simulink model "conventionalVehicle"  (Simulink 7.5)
settings: Solver=ode45  StartTime=0.0  StopTime=Tfinal  RelTol=1e-3
InitFcn:
  | t_Start=tic;
StopFcn:
  | t_elapsed=toc(t_Start);
  | fuel_cons=(1000*(fueltank_simple1_std(end,1)/fueltank_simple1_std(end,3)))/(chassis_simple4_std(end,2)/100000);
  | 
  | disp(' ')
  | disp(['Time Elapsed: ' num2str(round(100*t_elapsed)/100) 's'])
  | disp(['Fuel Consumption: ' num2str(round(1000*fuel_cons)/1000) 'L/100km'])
undefined symbols (not defined in the file or in its folder): computed_mass, DC, levelinit
libraries: simulink x10, simulink_extras x2
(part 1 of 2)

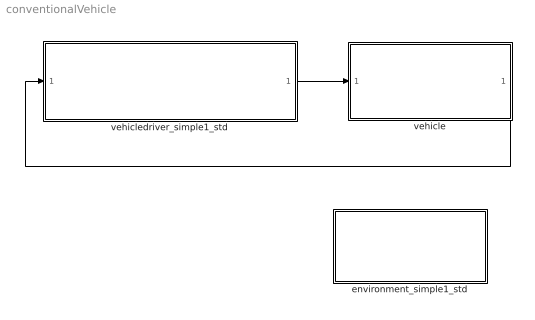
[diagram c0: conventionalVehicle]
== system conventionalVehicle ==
  environment_simple1_std : Subsystem  mask{Tamb=300, Pamb=101300}
      mask prompts: Tamb "Ambient Temperature [K]"; Pamb "Ambient Pressure [Pa]"
      mask help: Environment settings
  vehicle : Subsystem
  vehicledriver_simple1_std : Subsystem  mask{Kp_driver=0.5, Ki_driver=0.05, clutchtime=0.5, manualFlag=1, nog=5}
      mask prompts: Kp_driver "Proportional Gain"; Ki_driver "Integral Gain"; clutchtime "Gear change time"; manualFlag "Manual or automatic gearchange?"; nog "Number of gears"
      mask help: Driver model
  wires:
  vehicledriver_simple1_std/1(driver cmd out) -> vehicle/1(In1)
  vehicle/1(Out1) -> vehicledriver_simple1_std/1(vehicle fb in)

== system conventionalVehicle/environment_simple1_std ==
  Clock : Clock
  Constant : Constant  Value=Tamb  OutDataType=sfix(16)  OutScaling=2^0
  Constant1 : Constant  Value=Pamb  OutDataType=sfix(16)  OutScaling=2^0
  Mux : Mux  Inputs=3
  Mux1 : Mux  Inputs=3
  Mux2 : Mux  Inputs=5
  To Workspace : ToWorkspace  VariableName=environment_simple1_std  SampleTime=-1  SaveFormat=Array
  fric_time : Lookup  InputValues=DC.time  Table=DC.fric  OutDataType=sfix(16)  OutScaling=2^0
  gear_time : Lookup  InputValues=DC.time  Table=DC.gearnr  OutDataType=sfix(16)  OutScaling=2^0
  slope_x_time : Lookup  InputValues=DC.time  Table=DC.slope_x  OutDataType=sfix(16)  OutScaling=2^0
  slope_y_time : Lookup  InputValues=DC.time  Table=DC.slope_y  OutDataType=sfix(16)  OutScaling=2^0
  speed_ref_time : Lookup  InputValues=DC.time  Table=DC.speed  OutDataType=sfix(16)  OutScaling=2^0
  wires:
  Constant1/1 -> Mux/2, Mux2/5
  Constant/1 -> Mux/1, Mux2/4
  Mux/1 -> To Workspace/1
  Clock/1 -> speed_ref_time/1, gear_time/1, slope_x_time/1, slope_y_time/1, fric_time/1, Mux/3, Mux1/3  "t"
  Mux1/1 -> [drivecycle]
  gear_time/1 -> Mux1/2
  slope_x_time/1 -> Mux2/1
  slope_y_time/1 -> Mux2/2
  fric_time/1 -> Mux2/3
  Mux2/1 -> [environment]
  speed_ref_time/1 -> Mux1/1

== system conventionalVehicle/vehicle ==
  In1 : Inport  OutDataType=sfix(16)  OutScaling=2^0
  Bus Creator : BusCreator  Inputs=3
  Bus Creator1 : BusCreator  Inputs=1
  Bus Selector : BusSelector  OutputSignals=ice,clutch,gearbox,chassis
  Ground : Ground
  Terminator : Terminator
  chassis_simple4_std : Subsystem  InitFcn=computed_mass=calc_total_mass;
  clutch_simple1_std : Subsystem
  controller_conventional1_std : Subsystem  mask{pedalmap_pedal=[0 1], idleSpeed=78.5, pedalmap_speed=[0 700], pedalmap_torqueref=[0 0;350 350], maxTorque=400, maxBrakeTorque=40000}
      mask prompts: pedalmap_pedal "Pedal Map: Input pedalvector"; idleSpeed "Idle speed (rad/s)"; pedalmap_speed "Pedal Map: Input speedvector"; pedalmap_torqueref "Pedal Map: PedalMap (torqueref)"; maxTorque "Maximum torque reference (Nm)"; maxBrakeTorque "Maximum brake torque (Nm)"
      mask help: Main Controller
  engine_scalable1_std : Subsystem
  fueltank_simple1_std : Subsystem  mask{tanksize=68, level=100, fueldensity=737.2, Hf=44.6}
      mask prompts: tanksize "Size of fuel tank  [l]"; level "Level in tank [%]"; fueldensity "Fuel density [kg/m3]"; Hf "Specific Calorific Value [MJ/kg]"
      mask help: This is an ideal internal combustion engine component
  gearbox_manual1_std : Subsystem
  Out1 : Outport  OutDataType=sfix(16)  OutScaling=2^0
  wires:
  In1/1 -> controller_conventional1_std/1(driver cmd in)
  controller_conventional1_std/1(vehicle fb out) -> Out1/1
  gearbox_manual1_std/2(mech power out [Nm]) -> chassis_simple4_std/2(mech in [Nm])
  clutch_simple1_std/1(mech power out [Nm]) -> gearbox_manual1_std/2(mech power in [Nm])
  clutch_simple1_std/2(mech fb out [rad/s]) -> engine_scalable1_std/3(mech fb in [rad/s])
  engine_scalable1_std/2(mech out [Nm]) -> clutch_simple1_std/2(mech power in [Nm])
  fueltank_simple1_std/1(chem SCV out [MJ/kg]) -> engine_scalable1_std/2(chem SCV in [MJ/kg])
  engine_scalable1_std/3(chem fb out [kg/s]) -> fueltank_simple1_std/1(chem fb in [kg/s])
  gearbox_manual1_std/3(mech fb out [rad/s]) -> clutch_simple1_std/3(mech fb in [rad/s])
  chassis_simple4_std/2(mech fb out [rad/s]) -> gearbox_manual1_std/3(mech fb in [rad/s])
  Bus Creator/1 -> controller_conventional1_std/2(sensor in)
  controller_conventional1_std/2(cmd out) -> Bus Selector/1
  engine_scalable1_std/1(sensor out) -> Bus Creator/1
  gearbox_manual1_std/1(sensor out) -> Bus Creator/2
  chassis_simple4_std/1(sensor out) -> Bus Creator/3
  Bus Selector/1 -> engine_scalable1_std/1(cmd)  "<ice>"
  Bus Selector/2 -> clutch_simple1_std/1(cmd)  "<clutch>"
  Bus Selector/3 -> gearbox_manual1_std/1(cmd)  "<gearbox>"
  Bus Selector/4 -> chassis_simple4_std/1(cmd)  "<chassis>"
  chassis_simple4_std/3(el fb out [A]) -> Terminator/1
  Bus Creator1/1 -> chassis_simple4_std/3(el in [V])
  Ground/1 -> Bus Creator1/1  "voltage [V]"

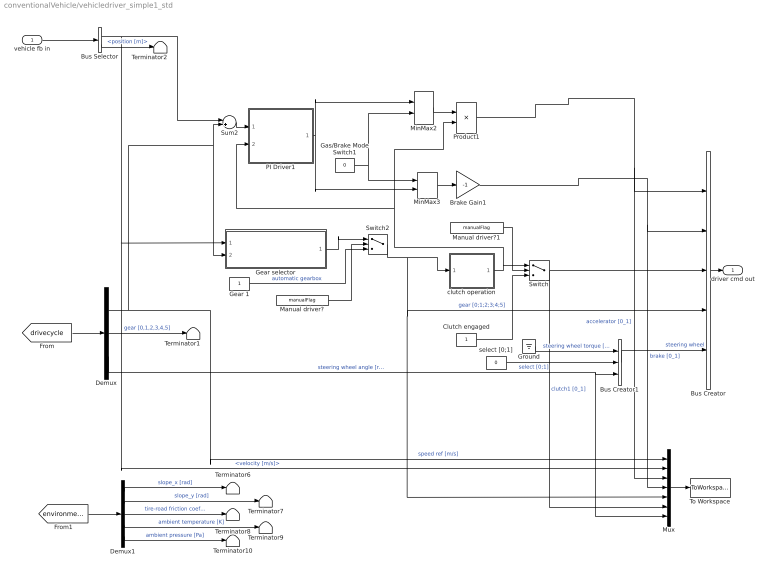
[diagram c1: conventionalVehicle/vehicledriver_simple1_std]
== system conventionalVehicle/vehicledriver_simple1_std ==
  vehicle fb in : Inport  OutDataType=sfix(16)  OutScaling=2^0
  Brake Gain1 : Gain  Gain=-1  ParameterDataType=sfix(16)  ParameterScaling=2^0  OutDataType=sfix(16)  OutScaling=2^0
  Bus Creator : BusCreator  Inputs=5
  Bus Creator1 : BusCreator  Inputs=3
  Bus Selector : BusSelector  OutputSignals=chassis.velocity [m/s],chassis.position [m]
  Clutch engaged : Constant  OutDataType=sfix(16)  OutScaling=2^0
  Demux : Demux  Outputs=3
  Demux1 : Demux  Outputs=5
  Gas/Brake Mode Switch1 : Constant  Value=0  OutDataType=sfix(16)  OutScaling=2^0
  Gear 1 : Constant  OutDataType=sfix(16)  OutScaling=2^0
  Gear selector : Subsystem
  Ground : Ground
  Manual driver? : Constant  Value=manualFlag  OutDataType=sfix(16)  OutScaling=2^0
  Manual driver?1 : Constant  Value=manualFlag  OutDataType=sfix(16)  OutScaling=2^0
  MinMax2 : MinMax  Function=max  Inputs=2  OutDataType=sfix(16)  OutScaling=2^0
  MinMax3 : MinMax  Inputs=2  OutDataType=sfix(16)  OutScaling=2^0
  Mux : Mux  Inputs=7
  PI Driver1 : Subsystem
  Product1 : Product  OutDataType=sfix(16)  OutScaling=2^0
  Sum2 : Sum  Inputs=-+  OutDataType=sfix(16)  OutScaling=2^0
  Switch : Switch  Criteria=u2 > Threshold
  Switch2 : Switch  Criteria=u2 > Threshold
  Terminator{1..2,6..10} (7 alike) : Terminator
  To Workspace : ToWorkspace  VariableName=vehicledriver_simple1_std  SampleTime=-1  SaveFormat=Array
  clutch operation : Subsystem
  select [0;1] : Constant  Value=0  OutDataType=sfix(16)  OutScaling=2^0
  driver cmd out : Outport  OutDataType=sfix(16)  OutScaling=2^0
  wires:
  Bus Selector/2 -> Terminator2/1  "<position [m]>"
  Bus Selector/1 -> Mux/2, Gear selector/1(Speed [m/s]), Sum2/1  "<velocity [m/s]>"
  vehicle fb in/1 -> Bus Selector/1
  Sum2/1 -> PI Driver1/1(PI input)
  Brake Gain1/1 -> Mux/4, Bus Creator/2  "brake [0_1]"
  PI Driver1/1(PI out) -> MinMax2/1, MinMax3/2
  MinMax3/1 -> Brake Gain1/1
  Gas/Brake Mode Switch1/1 -> MinMax2/2, MinMax3/1
  MinMax2/1 -> Product1/1
  Product1/1 -> Mux/3, Bus Creator/1  "accelerator [0_1]"
  Switch/1 -> Mux/6, Bus Creator/3  "clutch1 [0_1]"
  clutch operation/1(Clutch) -> Product1/2, PI Driver1/2(PI reset), Switch/1
  Switch2/1 -> Mux/5, Bus Creator/4, clutch operation/1(Gear)  "gear [0;1;2;3;4;5]"
  Bus Creator1/1 -> Bus Creator/5  "steering wheel"
  Mux/1 -> To Workspace/1
  Ground/1 -> Bus Creator1/1  "steering wheel torque [Nm]"
  Bus Creator/1 -> driver cmd out/1
  Manual driver?1/1 -> Switch/2
  Demux1/2 -> Terminator7/1  "slope_y [rad]"
  [environment] -> Demux1/1
  Demux1/3 -> Terminator8/1  "tire-road friction coefficient [-]"
  Demux1/1 -> Terminator6/1  "slope_x [rad]"
  Demux1/4 -> Terminator9/1  "ambient temperature [K]"
  Demux1/5 -> Terminator10/1  "ambient pressure [Pa]"
  Demux/2 -> Terminator1/1  "gear [0,1,2,3,4,5]"
  [drivecycle] -> Demux/1
  Demux/3 -> Bus Creator1/3, Mux/7  "steering wheel angle [rad]"
  Demux/1 -> Mux/1, Sum2/2, Gear selector/2(Speed ref [m/s])  "speed ref [m/s]"
  select [0;1]/1 -> Bus Creator1/2  "select [0;1]"
  Gear 1/1 -> Switch2/3  "automatic gearbox"
  Gear selector/1(Gear [0,1,2,3,4,5]) -> Switch2/1
  Manual driver?/1 -> Switch2/2
  Clutch engaged/1 -> Switch/3

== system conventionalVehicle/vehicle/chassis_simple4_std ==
  cmd : Inport  OutDataType=sfix(16)  OutScaling=2^0
  mech in [Nm] : Inport  Port=2  OutDataType=sfix(16)  OutScaling=2^0
  el in [V] : Inport  Port=3  OutDataType=sfix(16)  OutScaling=2^0
  chassis : Subsystem  mask{mass=??, nop=1, passengerweight=0, cargo=0, w_init=0, tirespec='215/45R16', e=0.01, Cd=0.3, Af=1.9, rho=1.29, finalgear=1}
      mask prompts: mass "Chassis Mass [kg]"; nop "Number of passengers"; passengerweight "Weight of avg. passenger (kg)"; cargo "Cargo load (kg)"; w_init "Initial velocity [rad/s]"; tirespec "Tire specification (ex: '205/55R16')"; e "Rolling resistance coeff rear"; Cd "Air resistance cd (-)"; Af "Air resistance frontal area (m2)"; rho "Air density (kg/m3)"; finalgear "Final gear"
      mask help: Chassis model template
      mask init:
      | r=tireradius(tirespec);
  local controller : Subsystem
  sensor out : Outport  OutDataType=sfix(16)  OutScaling=2^0
  mech fb out [rad/s] : Outport  Port=2  OutDataType=sfix(16)  OutScaling=2^0
  el fb out [A] : Outport  Port=3  OutDataType=sfix(16)  OutScaling=2^0
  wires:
  local controller/2(ctrl) -> chassis/1(ctrl)
  chassis/2(mech fb out [rad/s]) -> mech fb out [rad/s]/1
  mech in [Nm]/1 -> chassis/2(mech in [Nm])
  chassis/1(sensor out) -> local controller/2(sensor in)
  local controller/1(sensor out) -> sensor out/1
  cmd/1 -> local controller/1(cmd in)
  el in [V]/1 -> chassis/3(el in [V])
  chassis/3(el fb out [A]) -> el fb out [A]/1

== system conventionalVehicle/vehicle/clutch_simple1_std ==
  cmd : Inport  OutDataType=sfix(16)  OutScaling=2^0
  mech power in [Nm] : Inport  Port=2  OutDataType=sfix(16)  OutScaling=2^0
  mech fb in [rad/s] : Inport  Port=3  OutDataType=sfix(16)  OutScaling=2^0
  clutch : Subsystem  mask{mass=0, inertia=0.25, max_torque=500}
      mask prompts: mass "Component mass (kg)"; inertia "Clutch inertia (kgm^2)"; max_torque "Maximum clutch torque (Nm)"
  local controller : Subsystem
  mech power out [Nm] : Outport  OutDataType=sfix(16)  OutScaling=2^0
  mech fb out [rad/s] : Outport  Port=2  OutDataType=sfix(16)  OutScaling=2^0
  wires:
  mech power in [Nm]/1 -> clutch/2(mech power in [Nm])
  clutch/2(mech power out [Nm]) -> mech power out [Nm]/1
  mech fb in [rad/s]/1 -> clutch/3(mech fb in [rad/s])
  clutch/3(mech fb out [rad/s]) -> mech fb out [rad/s]/1
  cmd/1 -> local controller/1(cmd)
  local controller/1(ctrl) -> clutch/1(ctrl)
  clutch/1(sensor out) -> local controller/2(sensor in)

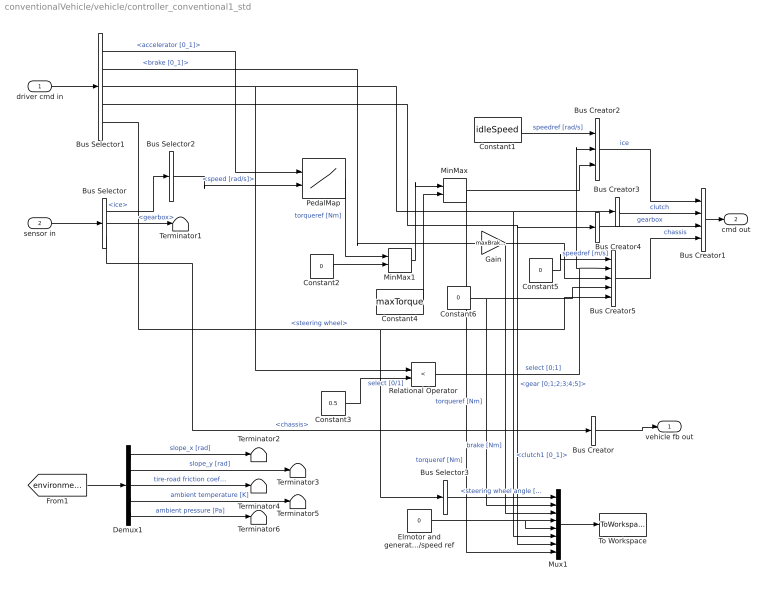
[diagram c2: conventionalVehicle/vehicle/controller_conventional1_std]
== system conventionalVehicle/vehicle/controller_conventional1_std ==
  driver cmd in : Inport  OutDataType=sfix(16)  OutScaling=2^0
  sensor in : Inport  Port=2  OutDataType=sfix(16)  OutScaling=2^0
  Bus Creator : BusCreator  Inputs=1
  Bus Creator1 : BusCreator
  Bus Creator2 : BusCreator  Inputs=3
  Bus Creator3 : BusCreator  Inputs=1
  Bus Creator4 : BusCreator  Inputs=1
  Bus Creator5 : BusCreator  Inputs=5
  Bus Selector : BusSelector  OutputSignals=ice,gearbox,chassis
  Bus Selector1 : BusSelector  OutputSignals=accelerator [0_1],brake [0_1],clutch1 [0_1],gear [0;1;2;3;4;5],steering wheel
  Bus Selector2 : BusSelector  OutputSignals=speed [rad/s]
  Bus Selector3 : BusSelector  OutputSignals=steering wheel angle [rad]
  Constant1 : Constant  Value=idleSpeed  OutDataType=sfix(16)  OutScaling=2^0
  Constant2 : Constant  Value=0  OutDataType=sfix(16)  OutScaling=2^0
  Constant3 : Constant  Value=0.5  OutDataType=sfix(16)  OutScaling=2^0
  Constant4 : Constant  Value=maxTorque  OutDataType=sfix(16)  OutScaling=2^0
  Constant5 : Constant  Value=0  OutDataType=sfix(16)  OutScaling=2^0
  Constant6 : Constant  Value=0  OutDataType=sfix(16)  OutScaling=2^0
  Demux1 : Demux  Outputs=5
  Elmotor and generator torque/speed ref : Constant  Value=0  OutDataType=sfix(16)  OutScaling=2^0
  Gain : Gain  Gain=maxBrakeTorque  ParameterDataType=sfix(16)  ParameterScaling=2^0  OutDataType=sfix(16)  OutScaling=2^0
  MinMax : MinMax  Inputs=2  OutDataType=sfix(16)  OutScaling=2^0
  MinMax1 : MinMax  Function=max  Inputs=2  OutDataType=sfix(16)  OutScaling=2^0
  Mux1 : Mux  Inputs=8
  PedalMap : Lookup2D  RowIndex=pedalmap_pedal  ColumnIndex=pedalmap_speed  Table=pedalmap_torqueref  OutDataType=sfix(16)  OutScaling=2^0
  Relational Operator : RelationalOperator  Operator=<
  Terminator{1..6} (6 alike) : Terminator
  To Workspace : ToWorkspace  VariableName=controller_conventional1_std  SampleTime=-1  SaveFormat=Array
  vehicle fb out : Outport  OutDataType=sfix(16)  OutScaling=2^0
  cmd out : Outport  Port=2  OutDataType=sfix(16)  OutScaling=2^0
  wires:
  Bus Selector2/1 -> PedalMap/2  "<speed [rad/s]>"
  Relational Operator/1 -> Bus Creator2/2, Bus Creator5/2  "select [0;1]"
  MinMax1/1 -> MinMax/1
  Constant4/1 -> MinMax/2
  Constant2/1 -> MinMax1/2
  PedalMap/1 -> MinMax1/1  "torqueref [Nm]"
  Constant3/1 -> Relational Operator/2  "select [0/1]"
  MinMax/1 -> Bus Creator2/3, Mux1/8  "torqueref [Nm]"
  Constant1/1 -> Bus Creator2/1  "speedref [rad/s]"
  Bus Creator2/1 -> Bus Creator1/1  "ice"
  Bus Creator1/1 -> cmd out/1
  Bus Creator/1 -> vehicle fb out/1
  Bus Selector/1 -> Bus Selector2/1  "<ice>"
  Bus Selector/2 -> Terminator1/1  "<gearbox>"
  Bus Selector/3 -> Bus Creator/1  "<chassis>"
  sensor in/1 -> Bus Selector/1
  driver cmd in/1 -> Bus Selector1/1
  Bus Creator3/1 -> Bus Creator1/2  "clutch"
  Bus Creator4/1 -> Bus Creator1/3  "gearbox"
  Gain/1 -> Bus Creator5/3, Mux1/3  "brake [Nm]"
  Bus Creator5/1 -> Bus Creator1/4  "chassis"
  Bus Selector1/1 -> PedalMap/1  "<accelerator [0_1]>"
  Bus Selector1/2 -> Gain/1  "<brake [0_1]>"
  Bus Selector1/3 -> Relational Operator/1, Bus Creator3/1, Mux1/6  "<clutch1 [0_1]>"
  Bus Selector1/5 -> Bus Creator5/5, Bus Selector3/1  "<steering wheel>"
  Bus Selector1/4 -> Bus Creator4/1, Mux1/7  "<gear [0;1;2;3;4;5]>"
  Mux1/1 -> To Workspace/1
  Bus Selector3/1 -> Mux1/1  "<steering wheel angle [rad]>"
  Constant5/1 -> Bus Creator5/1  "speedref [m/s]"
  Constant6/1 -> Bus Creator5/4, Mux1/2  "torqueref [Nm]"
  Elmotor and generator torque/speed ref/1 -> Mux1/4, Mux1/5
  Demux1/2 -> Terminator3/1  "slope_y [rad]"
  [environment] -> Demux1/1
  Demux1/3 -> Terminator4/1  "tire-road friction coefficient [-]"
  Demux1/1 -> Terminator2/1  "slope_x [rad]"
  Demux1/4 -> Terminator5/1  "ambient temperature [K]"
  Demux1/5 -> Terminator6/1  "ambient pressure [Pa]"

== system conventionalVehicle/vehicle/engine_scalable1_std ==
  cmd : Inport  OutDataType=sfix(16)  OutScaling=2^0
  chem SCV in [MJ/kg] : Inport  Port=2  OutDataType=sfix(16)  OutScaling=2^0
  mech fb in [rad/s] : Inport  Port=3  OutDataType=sfix(16)  OutScaling=2^0
  Model Info1 : simulink/Model-Wide Utilities/Model Info  SystemSampleTime=-1  InitialBlockCM=None  BlockCM=None  Frame=on  DisplayStringWithTags=This model level is fixed. Place parameters in the subsystem masks, not on the top level.  HorizontalTextAlignment=Left  LeftAlignmentValue=0.02  SourceBlockDiagram=conventionalVehicle  TagMaxNumber=20
  engine : Subsystem  mask{mass=0, inertia=??, N=??, S=??, B=??, e=??, k1=144000, k2=0.46, k3=0.00091, k4=0.075, p_me0g=??, PI=??}
      mask prompts: mass "Mass [kg]"; inertia "Flywheel inertia [kg*m/s2]"; N "Number of cylinders [-]"; S "Stroke [m]"; B "Bore [m]"; e "Thermal efficiency [-]"; k1 "Friction model coefficient 1 [Pa]"; k2 "Friction model coefficient 2 [-]"; k3 "Friction model coefficient 3 [s^2/m^2]"; k4 "Friction model coefficient 4 [m]"; p_me0g "Gas exchange loss [Pa]"; PI "Maximum boost ratio [-]"
      mask help: Internal combustion engine template model
  local controller : Subsystem  mask{N_c=??, S_c=??, B_c=??, e_c=??, k1_c=144000, k2_c=0.46, k3_c=0.00091, k4_c=0.075, p_me0g_c=??, PI_c=??, Kp_c=50, Ki_c=30, maxTorque=[177 4300], maxPower=[96 6100]}
      mask prompts: N_c "Number of cylinders [-]"; S_c "Stroke [m]"; B_c "Bore [m]"; e_c "Thermal efficiency [-]"; k1_c "Friction model coefficient 1 [Pa]"; k2_c "Friction model coefficient 2 [-]"; k3_c "Friction model coefficient 3 [s^2/m^2]"; k4_c "Friction model coefficient 4 [m]"; p_me0g_c "Gas exchange loss [Pa]"; PI_c "Maximum boost ratio [-]"; Kp_c "Speed controller Kp"; Ki_c "Speed controller Ki"; maxTorque "Max Torque at rpm (Nm rpm)"; maxPower "Max Power at rpm (kW rpm)"
      mask help: Local controller template for internal combustion engine
  sensor out : Outport  OutDataType=sfix(16)  OutScaling=2^0
  mech out [Nm] : Outport  Port=2  OutDataType=sfix(16)  OutScaling=2^0
  chem fb out [kg/s] : Outport  Port=3  OutDataType=sfix(16)  OutScaling=2^0
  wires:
  engine/2(mech power out [Nm]) -> mech out [Nm]/1
  mech fb in [rad/s]/1 -> engine/3(mech fb in [rad/s])
  engine/1(sensor out) -> local controller/2(sensor in)
  local controller/1(sensor out) -> sensor out/1
  cmd/1 -> local controller/1(cmd)
  local controller/2(ctrl) -> engine/1(ctrl)
  engine/3(chem fb out [kg/s]) -> chem fb out [kg/s]/1
  chem SCV in [MJ/kg]/1 -> engine/2(chem SCV in [MJ/kg])

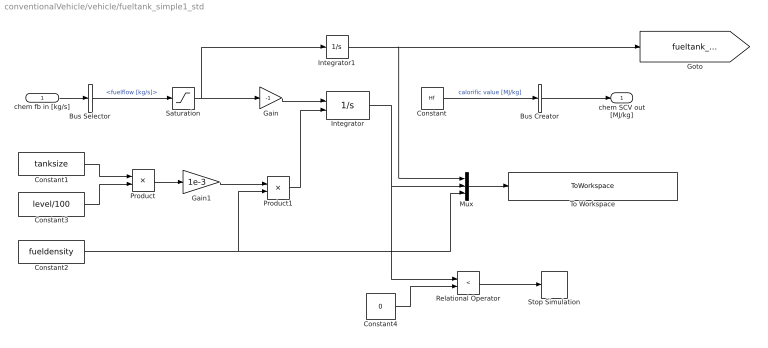
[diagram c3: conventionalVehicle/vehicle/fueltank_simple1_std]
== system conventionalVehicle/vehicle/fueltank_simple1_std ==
  chem fb in [kg/s] : Inport  OutDataType=sfix(16)  OutScaling=2^0
  Bus Creator : BusCreator  Inputs=1
  Bus Selector : BusSelector  OutputSignals=fuelflow [kg/s]
  Constant : Constant  Value=Hf  OutDataType=sfix(16)  OutScaling=2^0
  Constant1 : Constant  Value=tanksize  OutDataType=sfix(16)  OutScaling=2^0
  Constant2 : Constant  Value=fueldensity  OutDataType=sfix(16)  OutScaling=2^0
  Constant3 : Constant  Value=level/100  OutDataType=sfix(16)  OutScaling=2^0
  Constant4 : Constant  Value=0  OutDataType=sfix(16)  OutScaling=2^0
  Gain : Gain  Gain=-1  ParameterDataType=sfix(16)  ParameterScaling=2^0  OutDataType=sfix(16)  OutScaling=2^0
  Gain1 : Gain  Gain=1e-3  ParameterDataType=sfix(16)  ParameterScaling=2^0  OutDataType=sfix(16)  OutScaling=2^0
  Integrator : Integrator  InitialConditionSource=external  InitialCondition=levelinit
  Integrator1 : Integrator
  Mux : Mux  Inputs=3
  Product : Product  OutDataType=sfix(16)  OutScaling=2^0
  Product1 : Product  OutDataType=sfix(16)  OutScaling=2^0
  Relational Operator : RelationalOperator  Operator=<  LogicOutDataTypeMode=boolean  OutDataTypeStr=boolean
  Saturation : Saturate  UpperLimit=inf  LowerLimit=0
  Stop Simulation : Stop
  To Workspace : ToWorkspace  VariableName=fueltank_simple1_std  SampleTime=-1  SaveFormat=Array
  chem SCV out [MJ/kg] : Outport  OutDataType=sfix(16)  OutScaling=2^0
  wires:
  chem fb in [kg/s]/1 -> Bus Selector/1
  Constant/1 -> Bus Creator/1  "calorific value [MJ/kg]"
  Gain/1 -> Integrator/1
  Bus Selector/1 -> Saturation/1  "<fuelflow [kg/s]>"
  Mux/1 -> To Workspace/1
  Integrator1/1 -> [fueltank_weight_reduction], Mux/1
  Integrator/1 -> Mux/2, Relational Operator/1
  Bus Creator/1 -> chem SCV out [MJ/kg]/1
  Constant1/1 -> Product/1
  Constant3/1 -> Product/2
  Constant2/1 -> Mux/3, Product1/2
  Product/1 -> Gain1/1
  Product1/1 -> Integrator/2
  Gain1/1 -> Product1/1
  Constant4/1 -> Relational Operator/2
  Relational Operator/1 -> Stop Simulation/1
  Saturation/1 -> Gain/1, Integrator1/1

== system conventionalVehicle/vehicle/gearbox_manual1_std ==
  cmd : Inport  OutDataType=sfix(16)  OutScaling=2^0
  mech power in [Nm] : Inport  Port=2  OutDataType=sfix(16)  OutScaling=2^0
  mech fb in [rad/s] : Inport  Port=3  OutDataType=sfix(16)  OutScaling=2^0
  gearbox : Subsystem  mask{mass=0, nog=5, n_tragear_TabIp=[0 1 2 3 4 5], n_tragear_TabOp=[?? ?? ?? ?? ?? ??], gearinertia_tab=[0.005 0.006 0.008 0.013 0.021 0.031], geareff_tab=[?? ?? ?? ?? ?? ??], gearloss_tabIp=[0 722], gearloss_tab1=[?? ??], gearloss_tab2=[?? ??], gearloss_tab3=[?? ??], gearloss_tab4=[?? ??], gearloss_tab5=[?? ??], gearloss_tab0=[?? ??]}
      mask prompts: mass "Component mass [kg]"; nog "Number of gears"; n_tragear_TabIp "Gear number"; n_tragear_TabOp "Gear ratio"; gearinertia_tab "Gearbox inertia for each gear"; geareff_tab "Gear Efficiency table"; gearloss_tabIp "Pump and drag losses: Engine Speed [rad/s]"; gearloss_tab1 "Pump and drag losses: Torque Loss [Nm] (gear 1)"; gearloss_tab2 "Pump and drag losses: Torque Loss [Nm] (gear 2)"; gearloss_tab3 "Pump and drag losses: Torque Loss [Nm] (gear 3)"; gearloss_tab4 "Pump and drag losses: Torque Loss [Nm] (gear 4)"; gearloss_tab5 "Pump and drag losses: Torque Loss [Nm] (gear 5)"; gearloss_tab0 "Pump and drag losses: Torque Loss [Nm] (gear 0)"
  local controller : Subsystem
  sensor out : Outport  OutDataType=sfix(16)  OutScaling=2^0
  mech power out [Nm] : Outport  Port=2  OutDataType=sfix(16)  OutScaling=2^0
  mech fb out [rad/s] : Outport  Port=3  OutDataType=sfix(16)  OutScaling=2^0
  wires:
  gearbox/3(mech fb out [rad/s]) -> mech fb out [rad/s]/1
  mech power in [Nm]/1 -> gearbox/2(mech power in [Nm])
  gearbox/2(mech power out [Nm]) -> mech power out [Nm]/1
  mech fb in [rad/s]/1 -> gearbox/3(mech fb in [rad/s])
  cmd/1 -> local controller/1(cmd)
  local controller/2(ctrl) -> gearbox/1(ctrl)
  local controller/1(sensor out) -> sensor out/1
  gearbox/1(sensor out) -> local controller/2(sensor in)

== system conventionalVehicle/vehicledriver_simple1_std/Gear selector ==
  Speed [m/s] : Inport  OutDataType=sfix(16)  OutScaling=2^0
  Speed ref [m/s] : Inport  Port=2  OutDataType=sfix(16)  OutScaling=2^0
  Constant : Constant  Value=0  OutDataType=sfix(16)  OutScaling=2^0
  Gear3 : Relay  OnSwitchValue=25/3.6  OffSwitchValue=15/3.6  OutDataType=sfix(16)  OutScaling=2^0
  Gear4 : Relay  OnSwitchValue=40/3.6  OffSwitchValue=30/3.6  OutDataType=sfix(16)  OutScaling=2^0
  Gear5 : Relay  OnSwitchValue=70/3.6  OffSwitchValue=50/3.6  OutDataType=sfix(16)  OutScaling=2^0
  Gear6 : Relay  OnSwitchValue=100/3.6  OffSwitchValue=80/3.6  OutDataType=sfix(16)  OutScaling=2^0
  Saturation : Saturate  UpperLimit=nog  LowerLimit=0
  Sum : Sum  Inputs=6  OutDataType=sfix(16)  OutScaling=2^0
  Sum1 : Sum  Inputs=2  OutDataType=sfix(16)  OutScaling=2^0
  gear1 : Relay  OffSwitchValue=0  OutDataType=sfix(16)  OutScaling=2^0
  gear2 : Relay  OnSwitchValue=10/3.6  OffSwitchValue=2/3.6  OutDataType=sfix(16)  OutScaling=2^0
  Gear [0,1,2,3,4,5] : Outport  OutDataType=sfix(16)  OutScaling=2^0
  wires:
  Speed ref [m/s]/1 -> gear1/1
  Constant/1 -> Sum1/2
  Sum1/1 -> Saturation/1
  Sum/1 -> Sum1/1
  Gear5/1 -> Sum/5
  Gear4/1 -> Sum/4
  Gear3/1 -> Sum/3
  gear2/1 -> Sum/2
  gear1/1 -> Sum/1
  Speed [m/s]/1 -> Gear4/1, Gear3/1, gear2/1, Gear5/1, Gear6/1
  Gear6/1 -> Sum/6
  Saturation/1 -> Gear [0,1,2,3,4,5]/1

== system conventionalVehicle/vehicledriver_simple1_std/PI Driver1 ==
  PI input : Inport  OutDataType=sfix(16)  OutScaling=2^0
  PI reset : Inport  Port=2  OutDataType=sfix(16)  OutScaling=2^0
  Integrator : Integrator  ExternalReset=either  LimitOutput=on  UpperSaturationLimit=30  LowerSaturationLimit=0
  Ki : Gain  Gain=Ki_driver  ParameterDataType=sfix(16)  ParameterScaling=2^0  OutDataType=sfix(16)  OutScaling=2^0
  Kp : Gain  Gain=Kp_driver  ParameterDataType=sfix(16)  ParameterScaling=2^0  OutDataType=sfix(16)  OutScaling=2^0
  Saturation : Saturate  UpperLimit=1  LowerLimit=-1
  Sum : Sum  Inputs=|++  OutDataType=sfix(16)  OutScaling=2^0
  PI out : Outport  OutDataType=sfix(16)  OutScaling=2^0
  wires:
  PI input/1 -> Integrator/1, Kp/1
  Integrator/1 -> Ki/1
  Ki/1 -> Sum/2
  Sum/1 -> Saturation/1
  Saturation/1 -> PI out/1
  PI reset/1 -> Integrator/2
  Kp/1 -> Sum/1

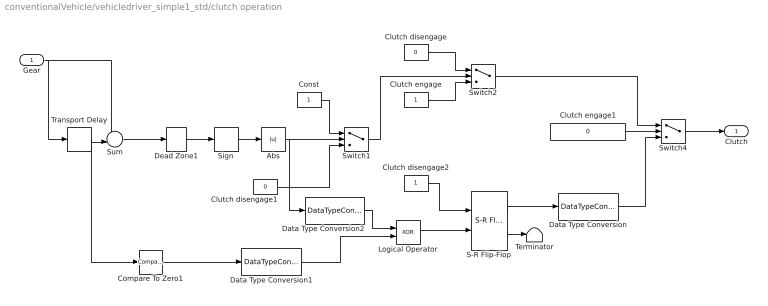
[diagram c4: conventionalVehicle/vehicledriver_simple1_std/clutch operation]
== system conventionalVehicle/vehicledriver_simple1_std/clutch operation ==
  Gear : Inport  OutDataType=sfix(16)  OutScaling=2^0
  Abs : Abs
  Clutch disengage : Constant  Value=0  OutDataType=sfix(16)  OutScaling=2^0
  Clutch disengage1 : Constant  Value=0  OutDataType=sfix(16)  OutScaling=2^0
  Clutch disengage2 : Constant  OutDataTypeMode=boolean  OutDataType=sfix(16)  OutScaling=2^0  OutDataTypeStr=boolean
  Clutch engage : Constant  OutDataType=sfix(16)  OutScaling=2^0
  Clutch engage1 : Constant  Value=0  OutDataType=sfix(16)  OutScaling=2^0
  Compare To Zero1 : simulink/Logic and Bit Operations/Compare To Zero  SystemSampleTime=-1  relop===  LogicOutDataTypeMode=uint8  ZeroCross=off
  Const : Constant  OutDataType=sfix(16)  OutScaling=2^0
  Data Type Conversion : DataTypeConversion  OutDataType=sfix(16)  OutScaling=2^0
  Data Type Conversion1 : DataTypeConversion  OutDataTypeMode=boolean  OutDataType=sfix(16)  OutScaling=2^0  OutDataTypeStr=boolean
  Data Type Conversion2 : DataTypeConversion  OutDataTypeMode=boolean  OutDataType=sfix(16)  OutScaling=2^0  OutDataTypeStr=boolean
  Dead Zone1 : DeadZone
  Logical Operator : Logic  Operator=XOR  AllPortsSameDT=off  OutDataTypeMode=boolean  OutDataTypeStr=boolean
  S-R Flip-Flop : simulink_extras/Flip Flops/S-R Flip-Flop  SystemSampleTime=-1  initial_condition=0
  Sign : Signum
  Sum : Sum  Inputs=-+|  OutDataType=sfix(16)  OutScaling=2^0
  Switch1 : Switch  Criteria=u2 ~= 0  Threshold=0.1
  Switch2 : Switch  Criteria=u2 ~= 0
  Switch4 : Switch  Criteria=u2 > Threshold  Threshold=0.5
  Terminator : Terminator
  Transport Delay : TransportDelay  DelayTime=clutchtime  BufferSize=4096
  Clutch : Outport  OutDataType=sfix(16)  OutScaling=2^0
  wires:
  Switch1/1 -> Switch2/2
  Clutch disengage/1 -> Switch2/1
  Clutch engage/1 -> Switch2/3
  Gear/1 -> Transport Delay/1, Sum/1
  Transport Delay/1 -> Sum/2, Compare To Zero1/1
  Sum/1 -> Dead Zone1/1
  Clutch disengage1/1 -> Switch1/3
  Dead Zone1/1 -> Sign/1
  Const/1 -> Switch1/1
  Switch4/1 -> Clutch/1
  Clutch engage1/1 -> Switch4/2
  Switch2/1 -> Switch4/1
  Sign/1 -> Abs/1
  Abs/1 -> Switch1/2, Data Type Conversion2/1
  Data Type Conversion/1 -> Switch4/3
  Compare To Zero1/1 -> Data Type Conversion1/1
  Data Type Conversion1/1 -> Logical Operator/2
  Data Type Conversion2/1 -> Logical Operator/1
  S-R Flip-Flop/1 -> Data Type Conversion/1
  Logical Operator/1 -> S-R Flip-Flop/2
  Clutch disengage2/1 -> S-R Flip-Flop/1
  S-R Flip-Flop/2 -> Terminator/1

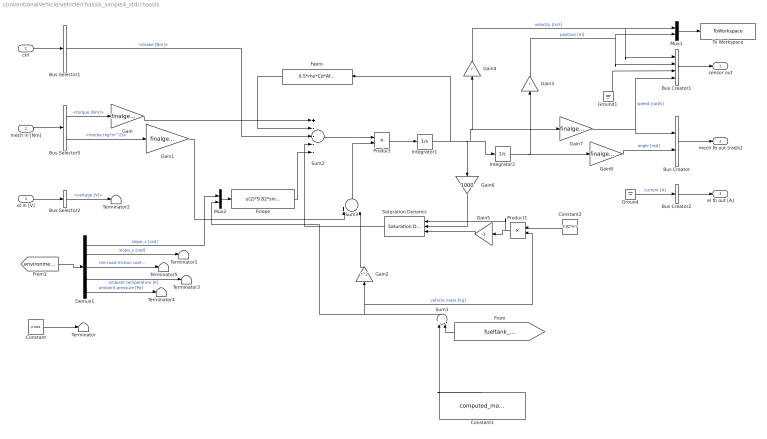
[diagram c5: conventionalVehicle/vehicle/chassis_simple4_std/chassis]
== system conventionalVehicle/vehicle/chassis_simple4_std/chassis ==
  ctrl : Inport  OutDataType=sfix(16)  OutScaling=2^0
  mech in [Nm] : Inport  Port=2  OutDataType=sfix(16)  OutScaling=2^0
  el in [V] : Inport  Port=3  OutDataType=sfix(16)  OutScaling=2^0
  Bus Creator : BusCreator  Inputs=2
  Bus Creator1 : BusCreator
  Bus Creator2 : BusCreator  Inputs=1
  Bus Selector1 : BusSelector  OutputSignals=brake [Nm]
  Bus Selector2 : BusSelector  OutputSignals=voltage [V]
  Bus Selector5 : BusSelector  OutputSignals=torque [Nm],inertia [kg*m^2]
  Constant : Constant  Value=mass  OutDataType=sfix(16)  OutScaling=2^0
  Constant1 : Constant  Value=computed_mass  OutDataType=sfix(16)  OutScaling=2^0
  Constant2 : Constant  Value=9.82*e*r  OutDataType=sfix(16)  OutScaling=2^0
  Demux1 : Demux  Outputs=5
  Faero : Fcn  Expr=0.5*rho*Cd*Af*u^2*r^3
  Fslope : Fcn  Expr=u(2)*9.82*sin(u(1))
  Gain : Gain  Gain=finalgear  ParameterDataType=sfix(16)  ParameterScaling=2^0  OutDataType=sfix(16)  OutScaling=2^0
  Gain1 : Gain  Gain=finalgear^2  ParameterDataType=sfix(16)  ParameterScaling=2^0  OutDataType=sfix(16)  OutScaling=2^0
  Gain2 : Gain  Gain=r^2  ParameterDataType=sfix(16)  ParameterScaling=2^0  OutDataType=sfix(16)  OutScaling=2^0
  Gain3 : Gain  Gain=r  ParameterDataType=sfix(16)  ParameterScaling=2^0  OutDataType=sfix(16)  OutScaling=2^0
  Gain4 : Gain  Gain=r  ParameterDataType=sfix(16)  ParameterScaling=2^0  OutDataType=sfix(16)  OutScaling=2^0
  Gain5 : Gain  Gain=-1  ParameterDataType=sfix(16)  ParameterScaling=2^0  OutDataType=sfix(16)  OutScaling=2^0
  Gain6 : Gain  Gain=1000  ParameterDataType=sfix(16)  ParameterScaling=2^0  OutDataType=sfix(16)  OutScaling=2^0
  Gain7 : Gain  Gain=finalgear  ParameterDataType=sfix(16)  ParameterScaling=2^0  OutDataType=sfix(16)  OutScaling=2^0
  Gain8 : Gain  Gain=finalgear  ParameterDataType=sfix(16)  ParameterScaling=2^0  OutDataType=sfix(16)  OutScaling=2^0
  Ground : Ground
  Ground1 : Ground
  Integrator1 : Integrator  InitialCondition=w_init
  Integrator2 : Integrator
  Mux1 : Mux  Inputs=2
  Mux2 : Mux  Inputs=2
  Product : Product  Inputs=*/  OutDataType=sfix(16)  OutScaling=2^0
  Product1 : Product  Inputs=**  OutDataType=sfix(16)  OutScaling=2^0
  Saturation Dynamic : simulink/Discontinuities/Saturation Dynamic  SystemSampleTime=-1  OutMin=[]  OutMax=[]  OutDataTypeStr=Inherit: Same as second input  OutDataType=sfix(16)  OutScaling=2^-10  DoSatur=off
  Sum1 : Sum  Inputs=+|-  OutDataType=sfix(16)  OutScaling=2^0
  Sum2 : Sum  Inputs=+----  OutDataType=sfix(16)  OutScaling=2^0
  Sum3 : Sum  OutDataType=sfix(16)  OutScaling=2^0
  Terminator{,1..5} (6 alike) : Terminator
  To Workspace : ToWorkspace  VariableName=chassis_simple4_std  SampleTime=-1  SaveFormat=Array
  sensor out : Outport  OutDataType=sfix(16)  OutScaling=2^0
  mech fb out [rad/s] : Outport  Port=2  OutDataType=sfix(16)  OutScaling=2^0
  el fb out [A] : Outport  Port=3  OutDataType=sfix(16)  OutScaling=2^0
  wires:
  Ground1/1 -> Bus Creator1/3
  Mux2/1 -> Fslope/1
  Bus Selector5/2 -> Gain1/1  "<inertia [kg*m^2]>"
  Bus Selector5/1 -> Gain/1  "<torque [Nm]>"
  Bus Creator/1 -> mech fb out [rad/s]/1
  mech in [Nm]/1 -> Bus Selector5/1
  Constant/1 -> Terminator/1
  Bus Creator1/1 -> sensor out/1
  Mux1/1 -> To Workspace/1
  ctrl/1 -> Bus Selector1/1
  Bus Selector2/1 -> Terminator2/1  "<voltage [V]>"
  el in [V]/1 -> Bus Selector2/1
  Bus Creator2/1 -> el fb out [A]/1
  Ground/1 -> Bus Creator2/1  "current [A]"
  Constant1/1 -> Sum1/1
  Sum1/1 -> Mux2/2, Gain2/1, Product1/2  "vehicle mass [kg]"
  [fueltank_weight_reduction] -> Sum1/2
  Demux1/2 -> Terminator1/1  "slope_y [rad]"
  [environment] -> Demux1/1
  Demux1/4 -> Terminator3/1  "ambient temperature [K]"
  Demux1/5 -> Terminator4/1  "ambient pressure [Pa]"
  Demux1/3 -> Terminator5/1  "tire-road friction coefficient [-]"
  Bus Selector1/1 -> Sum2/3  "<brake [Nm]>"
  Demux1/1 -> Mux2/1  "slope_x [rad]"
  Gain/1 -> Sum2/1
  Integrator1/1 -> Faero/1, Integrator2/1, Gain4/1, Gain7/1, Gain6/1
  Faero/1 -> Sum2/2
  Fslope/1 -> Sum2/5
  Integrator2/1 -> Gain3/1, Gain8/1
  Gain2/1 -> Sum3/2
  Gain1/1 -> Sum3/1
  Sum3/1 -> Product/2
  Product/1 -> Integrator1/1
  Sum2/1 -> Product/1
  Gain3/1 -> Mux1/2, Bus Creator1/2  "position [m]"
  Gain4/1 -> Mux1/1, Bus Creator1/1  "velocity [m/s]"
  Saturation Dynamic/1 -> Sum2/4
  Product1/1 -> Gain5/1, Saturation Dynamic/1
  Constant2/1 -> Product1/1
  Gain5/1 -> Saturation Dynamic/3
  Gain6/1 -> Saturation Dynamic/2
  Gain7/1 -> Bus Creator/1, Bus Creator1/4  "speed [rad/s]"
  Gain8/1 -> Bus Creator/2  "angle [rad]"

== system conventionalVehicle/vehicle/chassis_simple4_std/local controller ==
  cmd in : Inport  OutDataType=sfix(16)  OutScaling=2^0
  sensor in : Inport  Port=2  OutDataType=sfix(16)  OutScaling=2^0
  Bus Creator1 : BusCreator  Inputs=1
  Bus Creator2 : BusCreator  Inputs=2
  Bus Selector1 : BusSelector  OutputSignals=velocity [m/s],position [m]
  Bus Selector2 : BusSelector  OutputSignals=brake [Nm]
  sensor out : Outport  OutDataType=sfix(16)  OutScaling=2^0
  ctrl : Outport  Port=2  OutDataType=sfix(16)  OutScaling=2^0
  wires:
  Bus Selector2/1 -> Bus Creator1/1  "<brake [Nm]>"
  Bus Creator1/1 -> ctrl/1
  Bus Creator2/1 -> sensor out/1  "chassis"
  sensor in/1 -> Bus Selector1/1
  Bus Selector1/1 -> Bus Creator2/1  "<velocity [m/s]>"
  cmd in/1 -> Bus Selector2/1
  Bus Selector1/2 -> Bus Creator2/2  "<position [m]>"

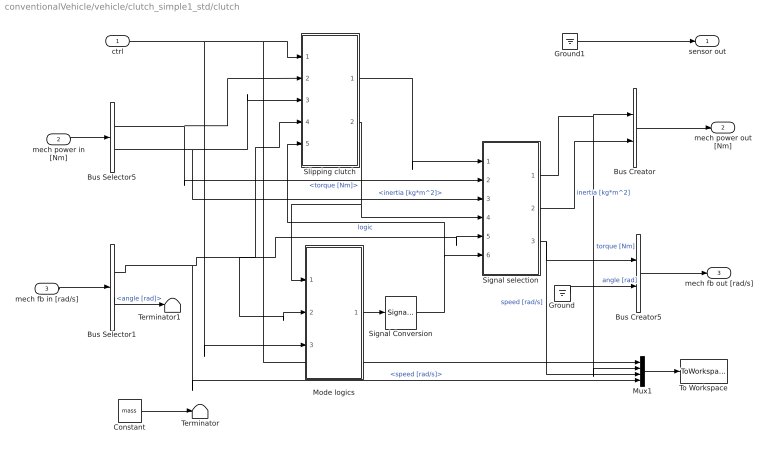
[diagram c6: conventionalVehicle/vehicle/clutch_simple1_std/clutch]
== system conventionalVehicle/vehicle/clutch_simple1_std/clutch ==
  ctrl : Inport  OutDataType=sfix(16)  OutScaling=2^0
  mech power in [Nm] : Inport  Port=2  OutDataType=sfix(16)  OutScaling=2^0
  mech fb in [rad/s] : Inport  Port=3  OutDataType=sfix(16)  OutScaling=2^0
  Bus Creator : BusCreator  Inputs=2
  Bus Creator5 : BusCreator  Inputs=2
  Bus Selector1 : BusSelector  OutputSignals=speed [rad/s],angle [rad]
  Bus Selector5 : BusSelector  OutputSignals=torque [Nm],inertia [kg*m^2]
  Constant : Constant  Value=mass  OutDataType=sfix(16)  OutScaling=2^0
  Ground : Ground
  Ground1 : Ground
  Mode logics : Subsystem
  Mux1 : Mux
  Signal Conversion : SignalConversion  ConversionOutput=Nonvirtual bus
  Signal selection : Subsystem
  Slipping clutch : Subsystem
  Terminator : Terminator
  Terminator1 : Terminator
  To Workspace : ToWorkspace  VariableName=clutch_simple1_std  SampleTime=-1  SaveFormat=Array
  sensor out : Outport  OutDataType=sfix(16)  OutScaling=2^0
  mech power out [Nm] : Outport  Port=2  OutDataType=sfix(16)  OutScaling=2^0
  mech fb out [rad/s] : Outport  Port=3  OutDataType=sfix(16)  OutScaling=2^0
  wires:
  Signal selection/3(speed) -> Bus Creator5/1, Mux1/3  "speed [rad/s]"
  Slipping clutch/1(torque) -> Signal selection/1(torque_out)
  Slipping clutch/2(speed) -> Signal selection/4(speed1), Mode logics/1(speed)
  Mode logics/1(logic) -> Signal Conversion/1
  Bus Selector5/2 -> Signal selection/3(inertia), Slipping clutch/3(inertia)  "<inertia [kg*m^2]>"
  Signal selection/1(torque) -> Bus Creator/1, Mux1/2  "torque [Nm]"
  Signal selection/2(inertia_out) -> Bus Creator/2  "inertia [kg*m^2]"
  ctrl/1 -> Mux1/1, Slipping clutch/1(Clutch_ctrl), Mode logics/3(clutch_ctrl)
  Ground/1 -> Bus Creator5/2  "angle [rad]"
  Bus Selector5/1 -> Signal selection/2(torque_in), Slipping clutch/2(torque_in)  "<torque [Nm]>"
  Bus Selector1/1 -> Signal selection/5(speed_fb), Slipping clutch/4(speed_fb), Mode logics/2(speed fb), Mux1/4  "<speed [rad/s]>"
  Constant/1 -> Terminator/1
  Bus Selector1/2 -> Terminator1/1  "<angle [rad]>"
  Mux1/1 -> To Workspace/1
  Signal Conversion/1 -> Slipping clutch/5(logic), Signal selection/6(logic)  "logic"
  Bus Creator/1 -> mech power out [Nm]/1
  mech power in [Nm]/1 -> Bus Selector5/1
  Bus Creator5/1 -> mech fb out [rad/s]/1
  mech fb in [rad/s]/1 -> Bus Selector1/1
  Ground1/1 -> sensor out/1

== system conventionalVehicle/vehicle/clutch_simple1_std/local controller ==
  cmd : Inport  OutDataType=sfix(16)  OutScaling=2^0
  sensor in : Inport  Port=2  OutDataType=sfix(16)  OutScaling=2^0
  Terminator : Terminator
  ctrl : Outport  OutDataType=sfix(16)  OutScaling=2^0
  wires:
  cmd/1 -> ctrl/1
  sensor in/1 -> Terminator/1

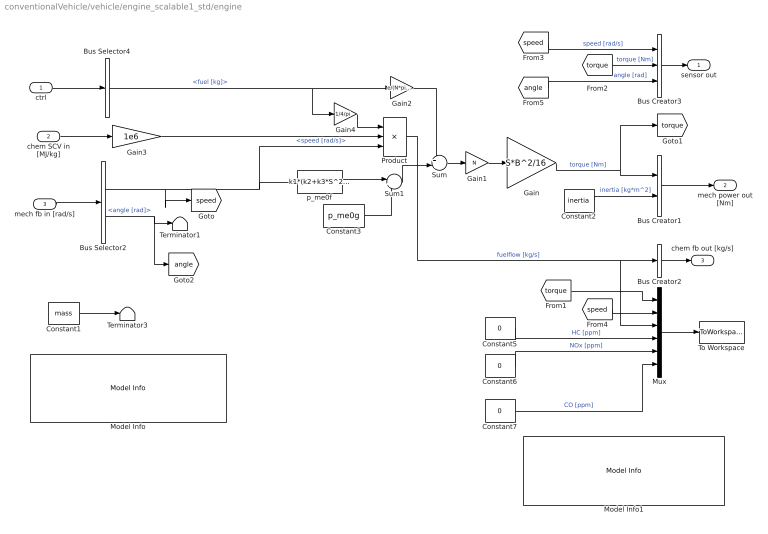
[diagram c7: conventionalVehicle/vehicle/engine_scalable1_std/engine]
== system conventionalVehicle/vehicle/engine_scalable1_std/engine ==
  ctrl : Inport  OutDataType=sfix(16)  OutScaling=2^0
  chem SCV in [MJ/kg] : Inport  Port=2  OutDataType=sfix(16)  OutScaling=2^0
  mech fb in [rad/s] : Inport  Port=3  OutDataType=sfix(16)  OutScaling=2^0
  Bus Creator1 : BusCreator  Inputs=2
  Bus Creator2 : BusCreator  Inputs=1
  Bus Creator3 : BusCreator  Inputs=3
  Bus Selector2 : BusSelector  OutputSignals=speed [rad/s],angle [rad]
  Bus Selector4 : BusSelector  OutputSignals=fuel [kg]
  Constant1 : Constant  Value=mass  OutDataType=sfix(16)  OutScaling=2^0
  Constant2 : Constant  Value=inertia  OutDataType=sfix(16)  OutScaling=2^0
  Constant3 : Constant  Value=p_me0g  OutDataType=sfix(16)  OutScaling=2^0
  Constant5 : Constant  Value=0  OutDataType=sfix(16)  OutScaling=2^0
  Constant6 : Constant  Value=0  OutDataType=sfix(16)  OutScaling=2^0
  Constant7 : Constant  Value=0  OutDataType=sfix(16)  OutScaling=2^0
  Gain : Gain  Gain=S*B^2/16  ParameterDataType=sfix(16)  ParameterScaling=2^0  OutDataType=sfix(16)  OutScaling=2^0
  Gain1 : Gain  Gain=N  ParameterDataType=sfix(16)  ParameterScaling=2^0  OutDataType=sfix(16)  OutScaling=2^0
  Gain2 : Gain  Gain=e/(N*pi*S*B^2/4)  ParameterDataType=sfix(16)  ParameterScaling=2^0  OutDataType=sfix(16)  OutScaling=2^0
  Gain3 : Gain  Gain=1e6  ParameterDataType=sfix(16)  ParameterScaling=2^0  OutDataType=sfix(16)  OutScaling=2^0
  Gain4 : Gain  Gain=1/4/pi  ParameterDataType=sfix(16)  ParameterScaling=2^0  OutDataType=sfix(16)  OutScaling=2^0
  Model Info : simulink/Model-Wide Utilities/Model Info  SystemSampleTime=-1  InitialBlockCM=None  BlockCM=None  Frame=on  DisplayStringWithTags=|  HorizontalTextAlignment=Left  LeftAlignmentValue=0.02  SourceBlockDiagram=conventionalVehicle  TagMaxNumber=20
      | Modified: %<ModifiedDate>
      | 
      | The nodes "ctrl" and "sensor out" must conform 
      | with the corresponding nodes of the local controller. 
      | The other nodes are fixed.
  Model Info1 : simulink/Model-Wide Utilities/Model Info  SystemSampleTime=-1  InitialBlockCM=None  BlockCM=None  Frame=on  DisplayStringWithTags=Your own comments!  HorizontalTextAlignment=Left  LeftAlignmentValue=0.02  SourceBlockDiagram=conventionalVehicle  TagMaxNumber=20
  Mux : Mux  Inputs=6
  Product : Product  Inputs=*/*  OutDataType=sfix(16)  OutScaling=2^0
  Sum : Sum  Inputs=+|-  OutDataType=sfix(16)  OutScaling=2^0
  Sum1 : Sum  Inputs=|++  OutDataType=sfix(16)  OutScaling=2^0
  Terminator1 : Terminator
  Terminator3 : Terminator
  To Workspace : ToWorkspace  VariableName=engine_scalable1_std  SampleTime=-1  SaveFormat=Array
  p_me0f : Fcn  Expr=k1*(k2+k3*S^2*u(1)^2)*PI*sqrt(k4/B)
  sensor out : Outport  OutDataType=sfix(16)  OutScaling=2^0
  mech power out [Nm] : Outport  Port=2  OutDataType=sfix(16)  OutScaling=2^0
  chem fb out [kg/s] : Outport  Port=3  OutDataType=sfix(16)  OutScaling=2^0
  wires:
  mech fb in [rad/s]/1 -> Bus Selector2/1
  Bus Creator1/1 -> mech power out [Nm]/1
  Bus Selector2/2 -> Terminator1/1, [angle]  "<angle [rad]>"
  Constant2/1 -> Bus Creator1/2  "inertia [kg*m^2]"
  Bus Selector2/1 -> [speed], p_me0f/1, Product/3  "<speed [rad/s]>"
  Bus Creator3/1 -> sensor out/1
  ctrl/1 -> Bus Selector4/1
  chem SCV in [MJ/kg]/1 -> Gain3/1
  Product/1 -> Bus Creator2/1, Mux/3  "fuelflow [kg/s]"
  Constant1/1 -> Terminator3/1
  Bus Creator2/1 -> chem fb out [kg/s]/1
  Mux/1 -> To Workspace/1
  [speed] -> Mux/2
  [speed] -> Bus Creator3/1  "speed [rad/s]"
  [torque] -> Bus Creator3/2  "torque [Nm]"
  [angle] -> Bus Creator3/3  "angle [rad]"
  Gain/1 -> Bus Creator1/1, [torque]  "torque [Nm]"
  [torque] -> Mux/1
  Gain1/1 -> Gain/1
  Sum/1 -> Gain1/1
  Sum1/1 -> Sum/2
  Constant3/1 -> Sum1/2
  p_me0f/1 -> Sum1/1
  Gain3/1 -> Product/2
  Bus Selector4/1 -> Gain2/1, Gain4/1  "<fuel [kg]>"
  Gain2/1 -> Sum/1
  Constant5/1 -> Mux/4  "HC [ppm]"
  Constant6/1 -> Mux/5  "NOx [ppm]"
  Constant7/1 -> Mux/6  "CO [ppm]"
  Gain4/1 -> Product/1

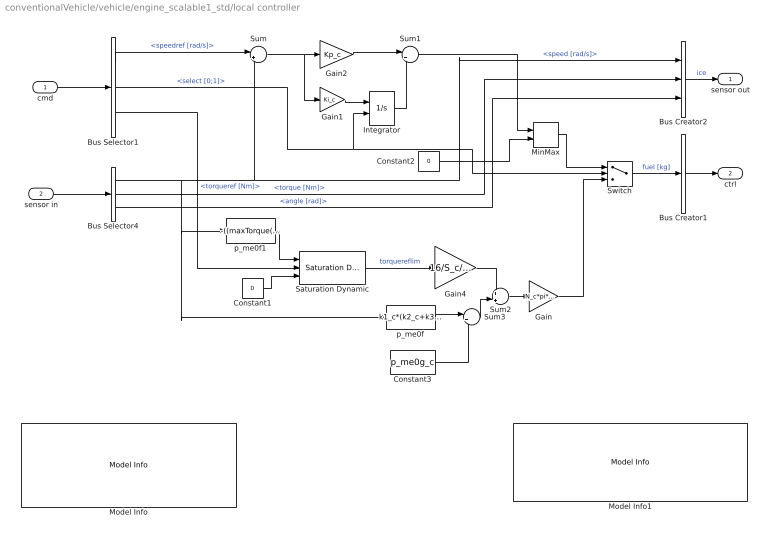
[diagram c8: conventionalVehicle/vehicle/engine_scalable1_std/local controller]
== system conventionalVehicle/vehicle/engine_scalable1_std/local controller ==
  cmd : Inport  OutDataType=sfix(16)  OutScaling=2^0
  sensor in : Inport  Port=2  OutDataType=sfix(16)  OutScaling=2^0
  Bus Creator1 : BusCreator  Inputs=1
  Bus Creator2 : BusCreator  Inputs=3
  Bus Selector1 : BusSelector  OutputSignals=speedref [rad/s],select [0;1],torqueref [Nm]
  Bus Selector4 : BusSelector  OutputSignals=speed [rad/s],torque [Nm],angle [rad]
  Constant1 : Constant  Value=0  OutDataType=sfix(16)  OutScaling=2^0
  Constant2 : Constant  Value=0  OutDataType=sfix(16)  OutScaling=2^0
  Constant3 : Constant  Value=p_me0g_c  OutDataType=sfix(16)  OutScaling=2^0
  Gain : Gain  Gain=N_c*pi*S_c*B_c^2/4/e_c  ParameterDataType=sfix(16)  ParameterScaling=2^0  OutDataType=sfix(16)  OutScaling=2^0
  Gain1 : Gain  Gain=Ki_c  ParameterDataType=sfix(16)  ParameterScaling=2^0  OutDataType=sfix(16)  OutScaling=2^0
  Gain2 : Gain  Gain=Kp_c  ParameterDataType=sfix(16)  ParameterScaling=2^0  OutDataType=sfix(16)  OutScaling=2^0
  Gain4 : Gain  Gain=16/S_c/(B_c^2)/N_c  ParameterDataType=sfix(16)  ParameterScaling=2^0  OutDataType=sfix(16)  OutScaling=2^0
  Integrator : Integrator  ExternalReset=either
  MinMax : MinMax  Function=max  Inputs=2  OutDataType=sfix(16)  OutScaling=2^0
  Model Info : simulink/Model-Wide Utilities/Model Info  SystemSampleTime=-1  InitialBlockCM=None  BlockCM=None  Frame=on  DisplayStringWithTags=|  HorizontalTextAlignment=Left  LeftAlignmentValue=0.02  SourceBlockDiagram=conventionalVehicle  TagMaxNumber=20
      | Modified: %<ModifiedDate>
      | The nodes "cmd" and "sensor out" are fixed.
      | The "select" signal defines whether the upper 
      | (=1) or lower (=0) signal is used.
      | The nodes "sensor in" and "ctrl", however, 
      | may be adjusted arbitrarily since the local 
      | controller is made specifically for a certain 
      | component model.
  Model Info1 : simulink/Model-Wide Utilities/Model Info  SystemSampleTime=-1  InitialBlockCM=None  BlockCM=None  Frame=on  DisplayStringWithTags=Your own comments!  HorizontalTextAlignment=Left  LeftAlignmentValue=0.02  SourceBlockDiagram=conventionalVehicle  TagMaxNumber=20
  Saturation Dynamic : simulink/Discontinuities/Saturation Dynamic  SystemSampleTime=-1  OutMin=[]  OutMax=[]  OutDataTypeStr=Inherit: Same as second input  OutDataType=sfix(16)  OutScaling=2^-10  DoSatur=off
  Sum : Sum  Inputs=|+-  OutDataType=sfix(16)  OutScaling=2^0
  Sum1 : Sum  Inputs=|++  OutDataType=sfix(16)  OutScaling=2^0
  Sum2 : Sum  Inputs=+|+  OutDataType=sfix(16)  OutScaling=2^0
  Sum3 : Sum  Inputs=|++  OutDataType=sfix(16)  OutScaling=2^0
  Switch : Switch  Threshold=0.5
  p_me0f : Fcn  Expr=k1_c*(k2_c+k3_c*S_c^2*u(1)^2)*PI_c*sqrt(k4_c/B_c)
  p_me0f1 : Fcn  Expr=-((maxTorque(1)-1000*maxPower(1)/(maxPower(2)/(60/2/pi)))/(((maxTorque(2)-maxPower(2))/(60/2/pi))^2))*(u[1]-maxTorque(2)/(60/2/pi))^2+maxTorque(1)
  sensor out : Outport  OutDataType=sfix(16)  OutScaling=2^0
  ctrl : Outport  Port=2  OutDataType=sfix(16)  OutScaling=2^0
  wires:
  Bus Creator1/1 -> ctrl/1
  Bus Creator2/1 -> sensor out/1  "ice"
  sensor in/1 -> Bus Selector4/1
  Bus Selector1/2 -> Switch/2, Integrator/2  "<select [0;1]>"
  Bus Selector1/1 -> Sum/1  "<speedref [rad/s]>"
  cmd/1 -> Bus Selector1/1
  Switch/1 -> Bus Creator1/1  "fuel [kg]"
  Bus Selector4/1 -> Sum/2, Bus Creator2/1, p_me0f/1, p_me0f1/1  "<speed [rad/s]>"
  Bus Selector4/2 -> Bus Creator2/2  "<torque [Nm]>"
  Bus Selector4/3 -> Bus Creator2/3  "<angle [rad]>"
  Gain1/1 -> Integrator/1
  Sum/1 -> Gain1/1, Gain2/1
  Gain2/1 -> Sum1/1
  Integrator/1 -> Sum1/2
  Gain4/1 -> Sum2/1
  Sum2/1 -> Gain/1
  Sum3/1 -> Sum2/2
  Constant3/1 -> Sum3/2
  p_me0f/1 -> Sum3/1
  Gain/1 -> Switch/3
  Saturation Dynamic/1 -> Gain4/1  "torquereflim"
  Bus Selector1/3 -> Saturation Dynamic/2  "<torqueref [Nm]>"
  Constant1/1 -> Saturation Dynamic/3
  p_me0f1/1 -> Saturation Dynamic/1
  MinMax/1 -> Switch/1
  Sum1/1 -> MinMax/1
  Constant2/1 -> MinMax/2

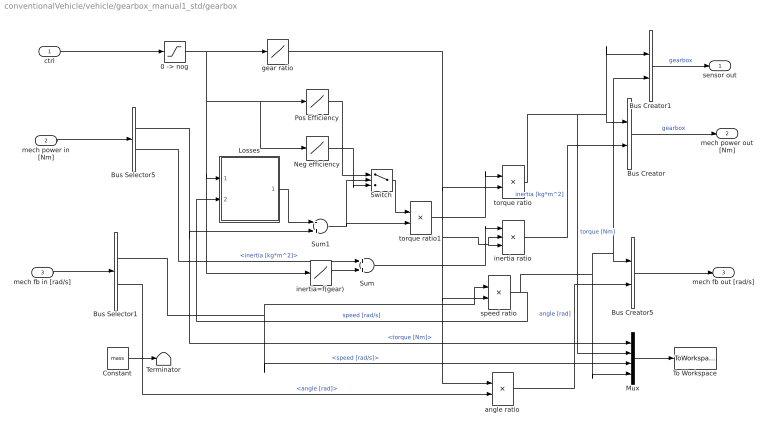
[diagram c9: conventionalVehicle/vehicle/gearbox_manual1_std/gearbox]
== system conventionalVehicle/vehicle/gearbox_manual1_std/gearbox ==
  ctrl : Inport  OutDataType=sfix(16)  OutScaling=2^0
  mech power in [Nm] : Inport  Port=2  OutDataType=sfix(16)  OutScaling=2^0
  mech fb in [rad/s] : Inport  Port=3  OutDataType=sfix(16)  OutScaling=2^0
  "0 -> nog" : Saturate  UpperLimit=n_tragear_TabIp(nog+1)  LowerLimit=0
  Bus Creator : BusCreator  Inputs=2
  Bus Creator1 : BusCreator  Inputs=2
  Bus Creator5 : BusCreator  Inputs=2
  Bus Selector1 : BusSelector  OutputSignals=speed [rad/s],angle [rad]
  Bus Selector5 : BusSelector  OutputSignals=torque [Nm],inertia [kg*m^2]
  Constant : Constant  Value=mass  OutDataType=sfix(16)  OutScaling=2^0
  Losses : Subsystem
  Mux : Mux
  Neg efficiency : Lookup  InputValues=n_tragear_TabIp  Table=1./geareff_tab  OutDataType=sfix(16)  OutScaling=2^0
  Pos Efficiency : Lookup  InputValues=n_tragear_TabIp  Table=geareff_tab  OutDataType=sfix(16)  OutScaling=2^0
  Sum : Sum  OutDataType=sfix(16)  OutScaling=2^0
  Sum1 : Sum  Inputs=-+  OutDataType=sfix(16)  OutScaling=2^0
  Switch : Switch  Threshold=0.1
  Terminator : Terminator
  To Workspace : ToWorkspace  VariableName=gearbox_manual1_std  SampleTime=-1  SaveFormat=Array
  angle ratio : Product  OutDataType=sfix(16)  OutScaling=2^0
  gear ratio : Lookup  InputValues=n_tragear_TabIp  Table=n_tragear_TabOp  OutDataType=sfix(16)  OutScaling=2^0
  inertia ratio : Product  Inputs=3  OutDataType=sfix(16)  OutScaling=2^0
  inertia=f(gear) : Lookup  InputValues=n_tragear_TabIp  Table=gearinertia_tab  OutDataType=sfix(16)  OutScaling=2^0
  speed ratio : Product  OutDataType=sfix(16)  OutScaling=2^0
  torque ratio : Product  OutDataType=sfix(16)  OutScaling=2^0
  torque ratio1 : Product  OutDataType=sfix(16)  OutScaling=2^0
  sensor out : Outport  OutDataType=sfix(16)  OutScaling=2^0
  mech power out [Nm] : Outport  Port=2  OutDataType=sfix(16)  OutScaling=2^0
  mech fb out [rad/s] : Outport  Port=3  OutDataType=sfix(16)  OutScaling=2^0
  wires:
  torque ratio/1 -> Bus Creator/1, Bus Creator1/1, Mux/2  "torque [Nm]"
  gear ratio/1 -> inertia ratio/3, inertia ratio/2, speed ratio/2, angle ratio/1, torque ratio/2
  Sum/1 -> inertia ratio/1
  Bus Selector1/1 -> Mux/3, speed ratio/1  "<speed [rad/s]>"
  inertia=f(gear)/1 -> Sum/2
  torque ratio1/1 -> torque ratio/1
  Neg efficiency/1 -> Switch/3
  Pos Efficiency/1 -> Switch/1
  Switch/1 -> torque ratio1/1
  Sum1/1 -> Switch/2, torque ratio1/2
  Losses/1(torque_loss) -> Sum1/1
  Bus Selector5/2 -> Sum/1  "<inertia [kg*m^2]>"
  Bus Selector5/1 -> Sum1/2, Mux/1  "<torque [Nm]>"
  "0 -> nog"/1 -> gear ratio/1, inertia=f(gear)/1, Losses/1(gear), Neg efficiency/1, Pos Efficiency/1
  angle ratio/1 -> Bus Creator5/2  "angle [rad]"
  speed ratio/1 -> Losses/2(speed), Bus Creator5/1, Bus Creator1/2, Mux/4  "speed [rad/s]"
  inertia ratio/1 -> Bus Creator/2  "inertia [kg*m^2]"
  Constant/1 -> Terminator/1
  Bus Selector1/2 -> angle ratio/2  "<angle [rad]>"
  Mux/1 -> To Workspace/1
  ctrl/1 -> "0 -> nog"/1
  Bus Creator1/1 -> sensor out/1  "gearbox"
  Bus Creator/1 -> mech power out [Nm]/1  "gearbox"
  mech power in [Nm]/1 -> Bus Selector5/1
  Bus Creator5/1 -> mech fb out [rad/s]/1
  mech fb in [rad/s]/1 -> Bus Selector1/1

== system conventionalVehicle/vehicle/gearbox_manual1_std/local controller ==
  cmd : Inport  OutDataType=sfix(16)  OutScaling=2^0
  sensor in : Inport  Port=2  OutDataType=sfix(16)  OutScaling=2^0
  Model Info : simulink/Model-Wide Utilities/Model Info  SystemSampleTime=-1  InitialBlockCM=None  BlockCM=None  Frame=on  DisplayStringWithTags=|  HorizontalTextAlignment=Left  LeftAlignmentValue=0.02  SourceBlockDiagram=conventionalVehicle  TagMaxNumber=20
      | Modified: %<ModifiedDate>
      | The nodes "cmd" and "sensor out" are fixed.
      | The "select" signal defines whether the upper 
      | (=1) or lower (=0) signal is used.
      | The nodes "sensor in" and "ctrl", however, 
      | may be adjusted arbitrarily since the local 
      | controller is made specifically for a certain 
      | component model.
  Model Info1 : simulink/Model-Wide Utilities/Model Info  SystemSampleTime=-1  InitialBlockCM=None  BlockCM=None  Frame=on  DisplayStringWithTags=Your own comments!  HorizontalTextAlignment=Left  LeftAlignmentValue=0.02  SourceBlockDiagram=conventionalVehicle  TagMaxNumber=20
  sensor out : Outport  OutDataType=sfix(16)  OutScaling=2^0
  ctrl : Outport  Port=2  OutDataType=sfix(16)  OutScaling=2^0
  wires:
  sensor in/1 -> sensor out/1
  cmd/1 -> ctrl/1

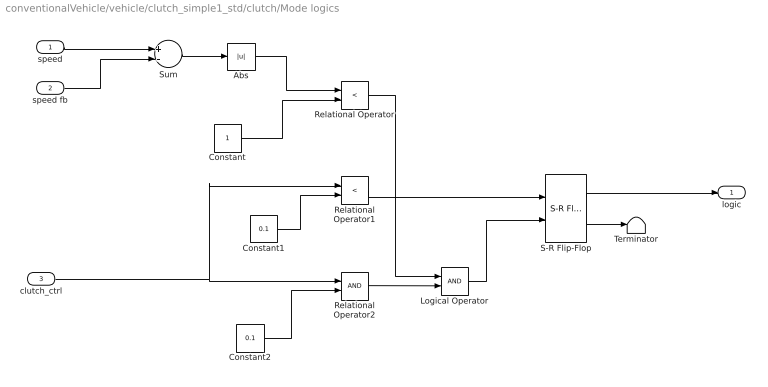
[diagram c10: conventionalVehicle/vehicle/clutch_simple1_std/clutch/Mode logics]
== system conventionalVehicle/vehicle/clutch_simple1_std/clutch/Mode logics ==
  speed : Inport  OutDataType=sfix(16)  OutScaling=2^0
  speed fb : Inport  Port=2  OutDataType=sfix(16)  OutScaling=2^0
  clutch_ctrl : Inport  Port=3  OutDataType=sfix(16)  OutScaling=2^0
  Abs : Abs
  Constant : Constant  OutDataType=sfix(16)  OutScaling=2^0
  Constant1 : Constant  Value=0.1  OutDataType=sfix(16)  OutScaling=2^0
  Constant2 : Constant  Value=0.1  OutDataType=sfix(16)  OutScaling=2^0
  Logical Operator : Logic  AllPortsSameDT=off
  Relational Operator : RelationalOperator  Operator=<
  Relational Operator1 : RelationalOperator  Operator=<
  Relational Operator2 : RelationalOperator
  S-R Flip-Flop : simulink_extras/Flip Flops/S-R Flip-Flop  SystemSampleTime=-1  initial_condition=0
  Sum : Sum  Inputs=+-  OutDataType=sfix(16)  OutScaling=2^0
  Terminator : Terminator
  logic : Outport  OutDataType=sfix(16)  OutScaling=2^0
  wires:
  S-R Flip-Flop/1 -> logic/1
  Relational Operator1/1 -> S-R Flip-Flop/1
  Constant1/1 -> Relational Operator1/2
  Relational Operator/1 -> Logical Operator/1
  Constant/1 -> Relational Operator/2
  Abs/1 -> Relational Operator/1
  Sum/1 -> Abs/1
  speed fb/1 -> Sum/2
  speed/1 -> Sum/1
  clutch_ctrl/1 -> Relational Operator1/1, Relational Operator2/1
  Constant2/1 -> Relational Operator2/2
  Relational Operator2/1 -> Logical Operator/2
  Logical Operator/1 -> S-R Flip-Flop/2
  S-R Flip-Flop/2 -> Terminator/1
